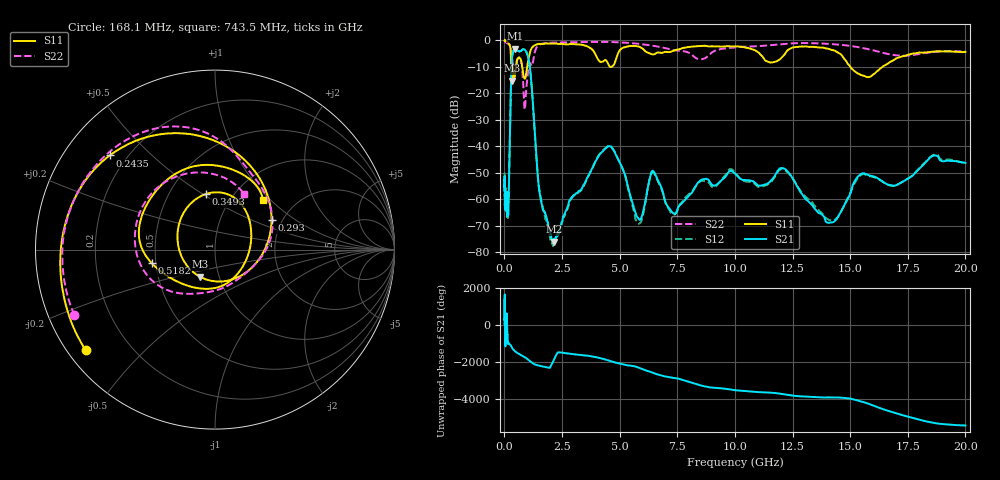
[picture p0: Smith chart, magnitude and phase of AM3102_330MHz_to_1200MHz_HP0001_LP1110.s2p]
! Date/Time: Tue, Sep 11, 2018 5:10 PM
! Network Analyzer: Agilent Technologies E8362B Rev: A.07.50.63
! Sweep from 0.010 to 20.000 GHz, 1601 Points, Sweep Type: LOG
! Power Supply: 4.949 V, 0.001 A
# Hz S DB R 50
!freq MagS11 AngS11 MagS21 AngS21 MagS12 AngS12 MagS22 AngS22
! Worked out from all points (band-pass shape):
!   1601 points, 10 MHz to 20 GHz, reference 50 ohm
!   highest |S21| = -3.11 dB at 471.2 MHz (marker M1); lowest = -76.1 dB at 2.165 GHz (marker M2)
!   |S21| within 3 dB of the highest: 338.9 MHz to 1.026 GHz (687.1 MHz wide, 101 % of centre)
!   lowest |S11| = -15.2 dB at 316.2 MHz (marker M3), VSWR 1.42, Z = 40.5 - j12.6 ohm
!   |S11| at or under -10 dB: 361.4 MHz to 504.2 MHz (142.8 MHz wide, 33 % of centre); 772.6 MHz to 987.5 MHz (215 MHz wide, 24.4 % of centre); 15.01 GHz to 16.4 GHz (1.393 GHz wide, 8.87 % of centre)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
!   |S22| runs from -26.1 to -0.3 dB; largest |S21 - S12| = 0.012
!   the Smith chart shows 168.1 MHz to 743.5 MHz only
!   S11 on the Smith chart (normalised r, x): 168.1 MHz: 0.05, -0.34; 243.5 MHz: 0.14, +0.38; 293 MHz: 1.76, +0.67; 349.3 MHz: 0.75, +0.51; 518.2 MHz: 0.47, -0.08; 743.5 MHz: 1.39, +0.91
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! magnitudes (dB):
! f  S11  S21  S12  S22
! 10 MHz  0.0  -53.1  -50.0  -0.3
! 35.55 MHz  0.0  -60.7  -61.7  -0.6
! 126.4 MHz  -0.4  -62.0  -64.3  -1.1
! 168.1 MHz  -0.8  -66.0  -63.1  -1.3
! 243.5 MHz  -2.1  -34.4  -34.5  -1.8
! 293 MHz  -9.0  -13.9  -13.9  -3.4
! 316.2 MHz  -15.2  -8.3  -8.3  -5.5
! 349.3 MHz  -10.1  -5.5  -5.6  -7.7
! 447.2 MHz  -13.7  -3.2  -3.2  -13.2
! 471.2 MHz  -12.6  -3.1  -3.1  -12.1
! 518.2 MHz  -8.9  -3.4  -3.5  -9.1
! 743.5 MHz  -8.3  -3.8  -3.8  -9.2
! 882.2 MHz  -14.4  -3.5  -3.6  -26.1
! 1.098 GHz  -5.0  -9.6  -9.6  -8.5
! 1.59 GHz  -1.3  -60.7  -60.0  -1.3
! 2.165 GHz  -1.2  -76.1  -76.1  -0.8
! 4.479 GHz  -8.5  -40.2  -40.1  -0.5
! 5.652 GHz  -2.1  -64.3  -65.7  -1.1
! 6.457 GHz  -5.3  -49.4  -50.0  -2.0
! 12.09 GHz  -5.9  -48.3  -48.7  -1.3
! 14.14 GHz  -3.4  -68.9  -68.0  -1.3
! 20 GHz  -4.4  -46.3  -46.6  -4.2
